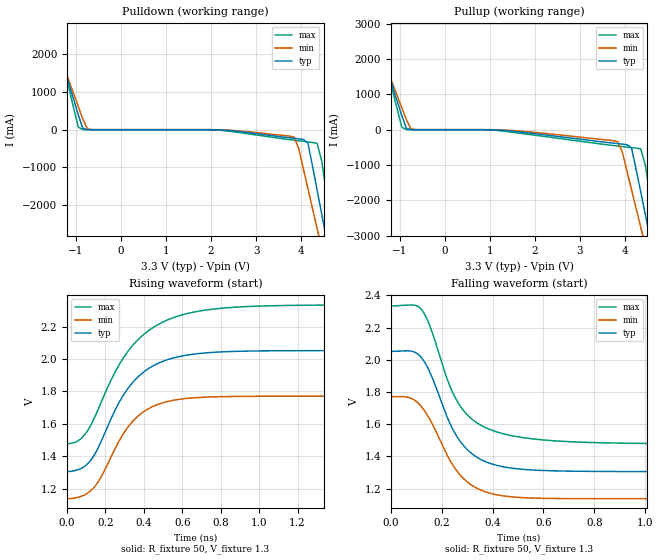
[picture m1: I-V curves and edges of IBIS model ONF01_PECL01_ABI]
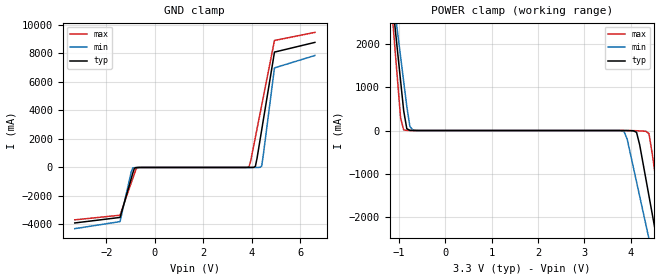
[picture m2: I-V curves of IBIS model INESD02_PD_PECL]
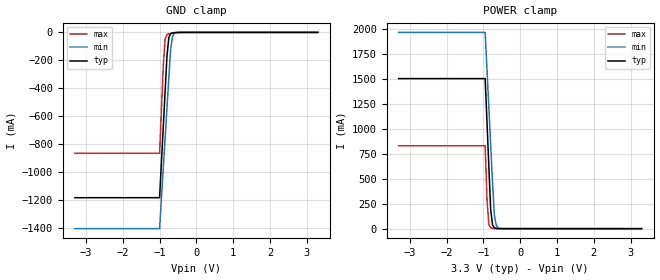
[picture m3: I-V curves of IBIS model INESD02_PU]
|   This file is an IBIS representation of the   |
|   Integrated Devices Technology, Inc.   |
|   ICS843004I-04   |
|   FEMTOCLOCKS CRYSTAL/LVCMOS-TO-3.3V LVPECL FREQUENCY SYNTHESIZER   |
[IBIS Ver]   4.1
[File name]   843004i_04_3v3.ibs
[File Rev]   1.0
[Date]   24 Dec 2008 | Last modified
|   24 Dec 2008 | Generated
[Source]   Originated at Integrated Devices Technology, Inc.
[Disclaimer]
IDT hereby grants the user of this IBIS model a non-exclusive,
nontransferable license to use this IBIS model under the following terms.
Before using this IBIS model, the user should read this license.
If the user does not accept these terms,  the IBIS model should be
returned to IDT within 30 days.
   The user is granted this license only to use the IBIS model and
is not granted rights to sell, load, rent, lease or license the IBIS
model in whole or in part, or in modified form to anyone other than
user. User may modify the IBIS model to suit its specific
applications but rights to derivative works and such modifications
shall belong to IDT.
   This IBIS model is provided on an "AS IS" basis and IDT makes
absolutely no warranty with respect to the information contained
herein. IDT DISCLAIMS AND CUSTOMER WAIVES ALL WARRANTIES, EXPRESS
OR IMPLIED, INCLUDING WARRANTIES OF MERCHANTABILITY OR FITNESS FOR
A PARTICULAR PURPOSE. The entire risk as to quality and performance
is with the Customer. ACCORDINGLY, IN NO EVENT SHALL THE COMPANY BE
LIABLE FOR ANY DAMAGES, WHETHER IN CONTRACT OR TORT,INCLUDING ANY
LOST PROFITS OR OTHER INCIDENTAL, CONSEQUENTIAL, EXEMPLARY, OR
PUNITIVE DAMAGES ARISING OUT OF THE USE OR APPLICATION OF THE IBIS
model provided in this package. Further, IDT reserves the right to
make changes without notice to any product herein to improve
reliability, function, or design. IDT does not convey any license
under patent rights or any other intellectual property rights,
including those of third parties.
   IDT is not obligated to provide maintenance or support
for the licensed IBIS model.
[Copyright]   Copyright 2004 byIntegrated Devices Technology, Inc.
[Component]   ICS843004I-04
[Manufacturer] Integrated Devices Technology, Inc.
[Package]
|TSSOP 24 Lead
|   typ   min   max
R_pkg   60.65m   52.4m   68.9m
L_pkg   1.989nH   1.431nH   2.547nH
C_pkg   0.314pF   0.254pF   0.374pF
[Pin]   signal_name   model_name   R_pin   L_pin   C_pin
1   nQ1   ONF01_PECL01_ABI   68.9m   2.547n   0.374p
2   Q1   ONF01_PECL01_ABI   65.6m   2.323n   0.350p
3   VCCO   POWER   62.3m   2.100n   0.326p
4   Q0   ONF01_PECL01_ABI   59.0m   1.877n   0.302p
5   nQ0   ONF01_PECL01_ABI   55.7m   1.654n   0.278p
6   MR   INESD02_PD_PECL   52.4m   1.431n   0.254p
7   F_SEL3   INESD02_PU   52.4m   1.431n   0.254p
8   NC   NC   55.7m   1.654n   0.278p
9   VCCA   POWER   59.0m   1.877n   0.302p
10  F_SEL0   INESD02_PU   62.3m   2.100n   0.326p
11  VCC   POWER   65.6m   2.323n   0.350p
12  F_SEL1   INESD02_PU   68.9m   2.547n   0.374p
13  XTAL_OUT   NC   68.9m   2.547n   0.374p
14  XTAL_IN   NC   65.6m   2.323n   0.350p
15  VEE   GND   62.3m   2.100n   0.326p
16  CLK   INESD02_PD_PECL   59.0m   1.877n   0.302p
17  INPUT_SEL   INESD02_PD   55.7m   1.654n   0.278p
18  F_SEL2   INESD02_PU   52.4m   1.431n   0.254p
19  VEE   GND   52.4m   1.431n   0.254p
20  nQ3   ONF01_PECL01_ABI   55.7m   1.654n   0.278p
21  Q3   ONF01_PECL01_ABI   59.0m   1.877n   0.302p
22  VCCO   POWER   62.3m   2.100n   0.326p
23  Q2   ONF01_PECL01_ABI   65.6m   2.323n   0.350p
24  nQ2   ONF01_PECL01_ABI   68.9m   2.547n   0.374p
[Diff Pin]  inv_pin  vdiff tdelay_typ tdelay_min  tdelay_max
2   1   NA   0   0   0
21   20   NA   0   0   0
23   24   NA   0   0   0
| Models and submodels in the file (4): ONF01_PECL01_ABI (Output_ECL), INESD02_PD_PECL (Input), INESD02_PU (Input), INESD02_PD (Input)
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[Model]   ONF01_PECL01_ABI
Model_type  Output_ECL
Polarity   Non-Inverting
Vmeas = 1.63
Rref = 50
Cref = 0
Vref = 1.3
|Variable  typ   min   max
C_comp   2p   1.5p   2.5p
[Voltage Range]   3.3   3.135   3.465
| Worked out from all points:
|   rising waveform, R_fixture 50, V_fixture 1.3: 20-80 % time 218ps typ, 193ps min, 263ps max; typ from 1.31 V to 2.05 V
|   falling waveform, R_fixture 50, V_fixture 1.3: 20-80 % time 134ps typ, 136ps min, 142ps max; typ from 2.05 V to 1.31 V
| Open source, no load
|  Voltage   I(typ)   I(min)   I(max)
[Pulldown]
-3.3V     9.786A     8.425A     12.06A
-1.667V   3.247A     2.986A     3.704A
-1.463V   2.432A     2.308A     2.661A
-952.6mV  398mA      618.5mA    68.87mA
-850.5mV  36.63mA    281.6mA    4.032mA
3.844V    -229.1mA   -195.7mA   -279.4mA
4.151V    -352.7mA   -1.559A    -324.9mA
4.355V    -1.599A    -2.62A     -360.9mA
4.559V    -2.871A    -3.681A    -1.635A
4.661V    -3.508A    -4.211A    -2.446A
4.763V    -4.144A    -4.742A    -3.257A
6.6V      -15.69A    -14.35A    -17.99A
[Pullup]
-3.3V     9.786A     8.425A     12.06A
-1.565V   2.839A     2.647A     3.182A
-952.6mV  398mA      618.5mA    68.87mA
-850.5mV  36.63mA    281.6mA    4.032mA
-646.4mV  229.3uA    964.8uA    177.5uA
3.844V    -394.4mA   -337mA     -463.1mA
4.151V    -517.8mA   -1.701A    -507.4mA
4.355V    -1.764A    -2.763A    -542.7mA
4.559V    -3.036A    -3.825A    -1.816A
4.661V    -3.672A    -4.355A    -2.626A
4.763V    -4.308A    -4.886A    -3.437A
6.6V      -15.79A    -14.46A    -18.06A
[Ramp]
|   typ   min   max
dV/dt_r   0.596/0.354n   0.506/0.311n   0.684/0.427n
dV/dt_f   0.599/0.219n   0.507/0.219n   0.690/0.252n
R_load =   50.0000
[Rising Waveform]
R_fixture = 50
V_fixture = 1.3   | VCC_typ - 2V
V_fixture_max = 1.465   | VCC_max - 2V
V_fixture_min = 1.135   | VCC_min - 2V
C_fixture = 0.0p
| Time   typ   min   max
0s        1.306V     1.138V     1.478V
67.2ps    1.321V     1.15V      1.503V
126ps     1.379V     1.19V      1.597V
176.4ps   1.489V     1.271V     1.731V
247.8ps   1.679V     1.442V     1.915V
338.1ps   1.85V      1.61V      2.079V
430.5ps   1.946V     1.698V     2.18V
554.4ps   2.007V     1.745V     2.255V
936.6ps   2.049V     1.77V      2.324V
1.999ns   2.052V     1.771V     2.333V
[Falling Waveform]
R_fixture = 50
V_fixture = 1.3   | VCC_typ - 2V
V_fixture_max = 1.465   | VCC_max - 2V
V_fixture_min = 1.135   | VCC_min - 2V
C_fixture = 0.0p
| Time   typ   min   max
0s        2.052V     1.771V     2.334V
73.5ps    2.055V     1.765V     2.34V
119.7ps   2.015V     1.711V     2.314V
151.2ps   1.932V     1.637V     2.221V
224.7ps   1.633V     1.399V     1.868V
268.8ps   1.503V     1.293V     1.723V
336ps     1.398V     1.205V     1.611V
434.7ps   1.338V     1.157V     1.544V
806.4ps   1.307V     1.138V     1.486V
1.999ns   1.306V     1.138V     1.478V
[Model]   INESD02_PD_PECL
Model_type  Input
Polarity   Non-Inverting
Vinl = 0.8V
Vinh = 2.0V
|   typ   min   max
C_comp   2pF   1.5pF   2.5pF
|   typ   min   max
[Voltage range]  3.3V   3.15V   3.45V
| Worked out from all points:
|   GND clamp passes 1 mA (typ) near -0.59 V on its own axis
|   POWER clamp passes 1 mA (typ) near -0.70 V on its own axis
[GND_clamp]
-3.3V     -3.894A    -4.294A    -3.674A
-1.434V   -3.506A    -3.799A    -3.352A
-974.8mV  -794.1mA   -331.5mA   -1.096A
-909.1mV  -407.1mA   -35.25mA   -774.3mA
-777.8mV  -10.55mA   -10.84mA   -133.1mA
-646.5mV  -1.912mA   -4.151mA   -2.665mA
3.884V    141.8uA    72.03uA    57.99mA
3.95V     342.2uA    75.94uA    423.8mA
4.146V    78.32mA    440.9uA    2.118A
4.409V    2.651A     112.4mA    4.38A
4.934V    8.093A     6.984A     8.908A
6.6V      8.773A     7.854A     9.475A
[POWER_clamp]
-3.3V     6.7A       6.327A     7.39A
-1.165V   3.23A      3.44A      2.951A
-1.031V   1.843A     2.286A     1.176A
-963.9mV  1.149A     1.709A     289.6mA
-896.9mV  456.5mA    1.133A     15.4mA
-695.9mV  792.2uA    10.73mA    555.6uA
3.861V    -556.7uA   -26.14mA   -39.45uA
4.129V    -41.85mA   -1.19A     -4.904mA
4.33V     -1.119A    -2.176A    -17.86mA
4.531V    -2.305A    -3.163A    -1.019A
4.732V    -3.492A    -4.151A    -2.536A
6.6V      -5.075A    -5.468A    -4.558A
[Model]   INESD02_PU
Model_type   Input
Polarity   Non-Inverting
Vinl = 0.80V
Vinh = 2.0V
|   typ   min   max
C_comp   2pF   1.5pF   2.5pF
|   typ   min   max
[Voltage range]  3.3V   3.15V   3.45V
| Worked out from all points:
|   GND clamp passes 1 mA (typ) near -0.56 V on its own axis
|   POWER clamp passes 1 mA (typ) near -0.61 V on its own axis
[GND_clamp]
|Voltage   I(typ)   I(min)   I(max)
-3.3V     -1.184A    -1.405A    -865.6mA
-1V       -1.184A    -1.405A    -865.6mA
-900mV    -678.5mA   -975.1mA   -244.1mA
-850mV    -426.2mA   -760.2mA   -46.92mA
-800mV    -174mA     -545.4mA   -16.17mA
-750mV    -37.03mA   -330.8mA   -9.981mA
-700mV    -9.767mA   -120.3mA   -7.122mA
-650mV    -3.616mA   -29.78mA   -4.922mA
-600mV    -1.7mA     -7.594mA   -3.115mA
-400mV    -123.9uA   -126uA     -173.9uA
3.3V      1.866nA    3.949uA    0A
[POWER_clamp]
|Voltage   I(typ)   I(min)   I(max)
-3.3V     1.506A     1.97A      832.1mA
-950mV    1.506A     1.97A      832.1mA
-900mV    1.063A     1.592A     287.2mA
-850mV    620.4mA    1.215A     41.77mA
-800mV    191.5mA    837.4mA    8.692mA
-750mV    37.69mA    460.1mA    3.262mA
-700mV    8.032mA    133.8mA    1.662mA
-650mV    2.005mA    32.58mA    840.1uA
-600mV    607uA      8.009mA    378.6uA
-450mV    33.11uA    139.8uA    23.88uA
3.3V      -71.13uA   -77.46uA   -62.11uA
